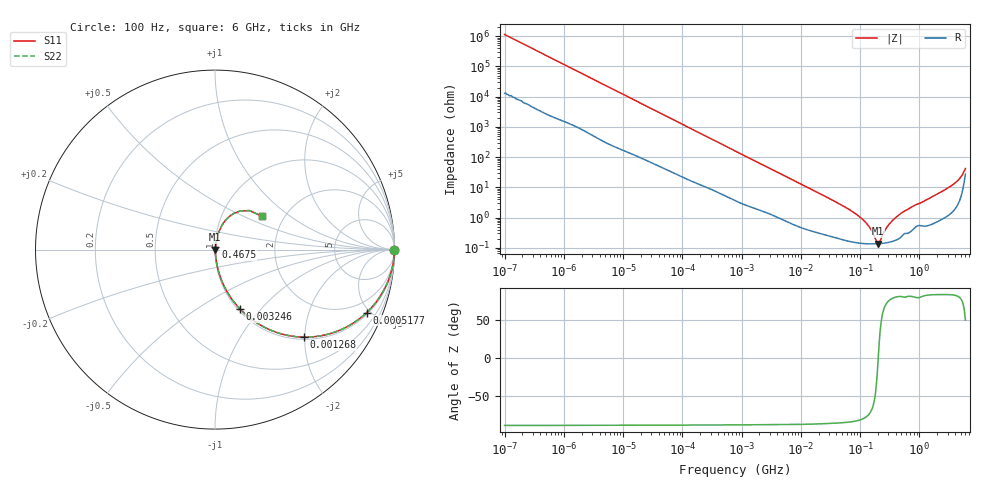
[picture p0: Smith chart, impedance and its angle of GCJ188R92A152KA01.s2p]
!Murata Part Number: GCJ188R92A152KA01
!These Parameters are Measured in Series Mode Connection
!Data Generated on Mar 13, 2026
!  o--ll--o
!Port1  Port2
!  o------o
!Operation Temp=25[degC], DC Bias Voltage=0[V]
!Freq. Start=100[Hz] Stop=6[GHz] 401[Steps]
# Hz S RI R 50
!Freq.(Hz) S11(Real) S11(Imag) S21(Real) S21(Imag) S12(Real) S12(Imag) S22(Real) S22(Imag)
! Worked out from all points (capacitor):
!   401 points, 100 Hz to 6 GHz, reference 50 ohm
!   read as one part in series: C = 1.39 nF near 109 Hz
!   lowest |Z| = 139 mohm at 199.7 MHz (marker M1)
!   series resonance near 202.9 MHz, so ESL is about 440 pH
!   S11 on the Smith chart (normalised r, x): 100 Hz: open; 517.7 kHz: 1.11, -4.78; 1.268 MHz: 1.05, -1.97; 3.246 MHz: 1.02, -0.78; 467.5 MHz: 1.00, +0.03; 6 GHz: 1.55, +0.64
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100  1 -8.77e-05  1e-06 8.77e-05  1e-06 8.77e-05  1 -8.77e-05
131  1 -0.000115  1.4e-06 0.000115  1.4e-06 0.000115  1 -0.000115
2008  1 -0.00172  2.73e-05 0.00172  2.73e-05 0.00172  1 -0.00172
40335  0.9983 -0.0336  0.0017 0.0336  0.0017 0.0336  0.9983 -0.0336
161617  0.9802 -0.1298  0.0198 0.1298  0.0198 0.1298  0.9802 -0.1298
517687  0.8454 -0.3505  0.1546 0.3505  0.1546 0.3505  0.8454 -0.3505
774597  0.7159 -0.4398  0.2841 0.4398  0.2841 0.4398  0.7159 -0.4398
1267578  0.4934 -0.4877  0.5066 0.4877  0.5066 0.4877  0.4934 -0.4877
3245845  0.1408 -0.3324  0.8592 0.3324  0.8592 0.3324  0.1408 -0.3324
6075234  0.0491 -0.2  0.9509 0.2  0.9509 0.2  0.0491 -0.2
1.555665e7  0.0104 -0.0824  0.9896 0.0824  0.9896 0.0824  0.0104 -0.0824
5.211241e7  0.0024 -0.024  0.9976 0.024  0.9976 0.024  0.0024 -0.024
9.753859e7  0.00155 -0.0107  0.9985 0.0107  0.9985 0.0107  0.00155 -0.0107
1.395531e8  0.00138 -0.00512  0.9986 0.00512  0.9986 0.00512  0.00138 -0.00512
1.996653e8  0.00137 -0.000212  0.9986 0.000212  0.9986 0.000212  0.00137 -0.000212
2.183701e8  0.00139 0.000988  0.9986 -0.000988  0.9986 -0.000988  0.00139 0.000988
2.61201e8  0.00145 0.00343  0.9985 -0.00343  0.9985 -0.00343  0.00145 0.00343
3.124326e8  0.00157 0.00598  0.9984 -0.00598  0.9984 -0.00598  0.00157 0.00598
4.674818e8  0.00226 0.0127  0.9977 -0.0127  0.9977 -0.0127  0.00226 0.0127
3.8344e9  0.0327 0.1232  0.9673 -0.1232  0.9673 -0.1232  0.0327 0.1232
5.016141e9  0.0833 0.1874  0.9167 -0.1874  0.9167 -0.1874  0.0833 0.1874
6e9  0.261 0.1858  0.739 -0.1858  0.739 -0.1858  0.261 0.1858
